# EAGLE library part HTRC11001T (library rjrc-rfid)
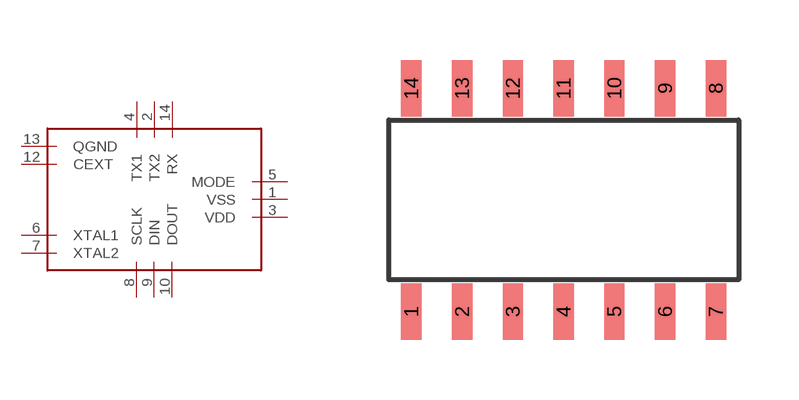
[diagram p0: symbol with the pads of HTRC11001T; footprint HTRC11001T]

Designator prefix -

## HTRC11001T  [HTRC11001T]
1  VSS
2  TX2
3  VDD
4  TX1
5  MODE
6  XTAL1
7  XTAL2
8  SCLK
9  DIN
10  DOUT
12  CEXT
13  QGND
14  RX

## Footprint HTRC11001T (pad centres in mm)
smd 0.508 x 1.422: 1 -3.81,-2.794; 2 -2.54,-2.794; 3 -1.27,-2.794; 4 0,-2.794; 5 1.27,-2.794; 6 2.54,-2.794; 7 3.81,-2.794; 8 3.81,2.794; 9 2.54,2.794; 10 1.27,2.794; 11 0,2.794; 12 -1.27,2.794; 13 -2.54,2.794; 14 -3.81,2.794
